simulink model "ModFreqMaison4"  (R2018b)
settings: Solver=FixedStepAuto  StartTime=0.0  StopTime=10  FixedStep=1e-5  RelTol=1e-4
libraries: simulink x1, commsynccomp2 x1, commrandsrc2 x1

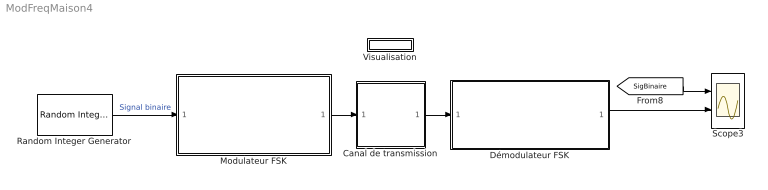
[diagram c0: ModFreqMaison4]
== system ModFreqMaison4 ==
  Canal de transmission : Subsystem
  Démodulateur FSK : Subsystem
  Modulateur FSK : Subsystem
  Random Integer Generator : commrandsrc2/Random Integer Generator  mul=4  seed=37  Ts=1  frameBased=off  sampPerFrame=1  orient=off  outDataType=double
  Scope3 : Scope  NumInputPorts=2
  Visualisation : Subsystem
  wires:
  [SigBinaire] -> Scope3/1
  Random Integer Generator/1 -> Modulateur FSK/1(Signal binaire)  "Signal binaire"
  Modulateur FSK/1(Signal Modulé FSK) -> Canal de transmission/1(In1)
  Démodulateur FSK/1(Signal démodulé) -> Scope3/2
  Canal de transmission/1(Out1) -> Démodulateur FSK/1(Signal modulé reçu)

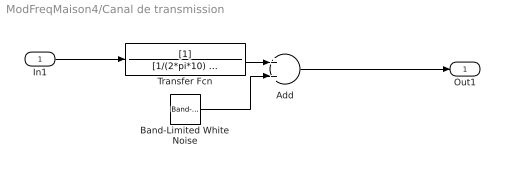
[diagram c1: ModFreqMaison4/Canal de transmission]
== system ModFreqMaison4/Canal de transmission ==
  In1 : Inport
  Add : Sum
  Band-Limited White Noise : simulink/Sources/Band-Limited White Noise  Cov=[0.002]  Ts=1  seed=[23341]
  Transfer Fcn : TransferFcn  Denominator=[1/(2*pi*10) 1]
  Out1 : Outport
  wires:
  Add/1 -> Out1/1
  Band-Limited White Noise/1 -> Add/2
  Transfer Fcn/1 -> Add/1
  In1/1 -> Transfer Fcn/1

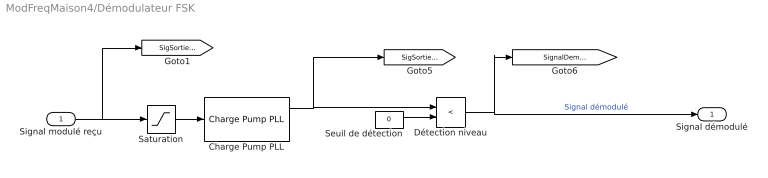
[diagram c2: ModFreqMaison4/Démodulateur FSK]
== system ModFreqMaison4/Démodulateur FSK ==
  Signal modulé reçu : Inport
  Charge Pump PLL : commsynccomp2/Charge Pump PLL  Fn=[2*pi*1]  Fd="[1   2*pi*1]"  Kvco=4  Fc=10  Ph=0  Ac=2
  Détection niveau : RelationalOperator  Operator=<  OutDataTypeStr=boolean
  Saturation : Saturate  UpperLimit=2  LowerLimit=-2
  Seuil de détection : Constant  Value=0
  Signal démodulé : Outport
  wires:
  Charge Pump PLL/1 -> Détection niveau/1, [SigSortiePLL]
  Seuil de détection/1 -> Détection niveau/2
  Détection niveau/1 -> Signal démodulé/1, [SignalDemodule]  "Signal démodulé"
  Saturation/1 -> Charge Pump PLL/1
  Signal modulé reçu/1 -> [SigSortieCanal], Saturation/1

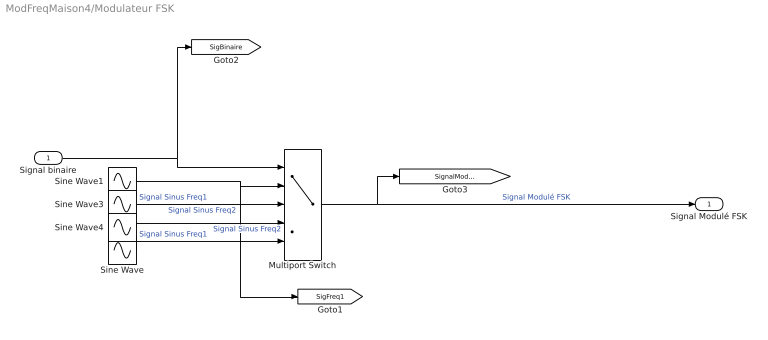
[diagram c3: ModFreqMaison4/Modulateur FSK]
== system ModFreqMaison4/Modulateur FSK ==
  Signal binaire : Inport
  Multiport Switch : MultiPortSwitch  DataPortOrder=Specify indices  Inputs=4  DataPortIndices={0,1,2,3}
  Sine Wave : Sin  Frequency=2*pi*35  Samples=25  SampleTime=0.001
  Sine Wave1 : Sin  Frequency=2*pi*5  Samples=50  SampleTime=0.001
  Sine Wave3 : Sin  Frequency=2*pi*15  Samples=25  SampleTime=0.001
  Sine Wave4 : Sin  Frequency=2*pi*25  Samples=50  SampleTime=0.001
  Signal Modulé FSK : Outport
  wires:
  Multiport Switch/1 -> Signal Modulé FSK/1, [SignalModuleFSK]  "Signal Modulé FSK"
  Signal binaire/1 -> Multiport Switch/1, [SigBinaire]
  Sine Wave1/1 -> [SigFreq1], Multiport Switch/2  "Signal Sinus Freq2"
  Sine Wave/1 -> Multiport Switch/5  "Signal Sinus Freq1"
  Sine Wave4/1 -> Multiport Switch/4  "Signal Sinus Freq2"
  Sine Wave3/1 -> Multiport Switch/3  "Signal Sinus Freq1"

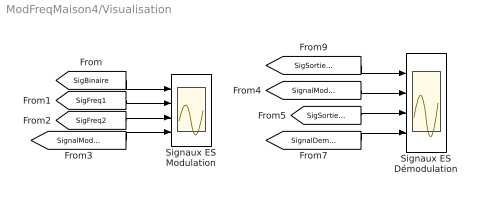
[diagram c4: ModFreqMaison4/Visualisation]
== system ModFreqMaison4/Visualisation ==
  Signaux ES Démodulation : Scope  NumInputPorts=4
  Signaux ES Modulation : Scope  NumInputPorts=4
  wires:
  [SignalModuleFSK] -> Signaux ES Démodulation/2
  [SignalModuleFSK] -> Signaux ES Modulation/4
  [SigFreq2] -> Signaux ES Modulation/3
  [SigFreq1] -> Signaux ES Modulation/2
  [SigBinaire] -> Signaux ES Modulation/1
  [SignalDemodule] -> Signaux ES Démodulation/4
  [SigSortiePLL] -> Signaux ES Démodulation/3
  [SigSortieCanal] -> Signaux ES Démodulation/1
